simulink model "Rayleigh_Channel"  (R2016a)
settings: Solver=ode3  StartTime=0.0  StopTime=6  FixedStep=1/5000000  RelTol=1e-3
libraries: commchan3 x1

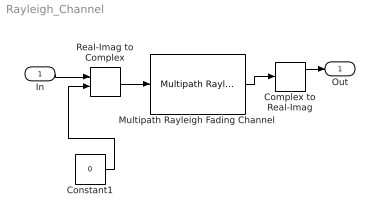
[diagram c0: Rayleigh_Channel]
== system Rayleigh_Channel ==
  In : Inport
  Complex to Real-Imag : ComplexToRealImag
  Constant1 : Constant  Value=0  SampleTime=1/5000000
  Multipath Rayleigh Fading Channel : commchan3/Multipath Rayleigh Fading Channel  maxDopplerShift=1  spectrumType=Jakes  sigmaGaussian=1/sqrt(2)  coeffRounded=[1 -1.72 0.785]  freqMinMaxRJakes=[0 1]  freqMinMaxAJakes=[0 1]  sigmaGaussian1=1/sqrt(2)  sigmaGaussian2=1/sqrt(2)  centerFreqGaussian1=0.0  centerFreqGaussian2=0.0  gainGaussian1=0.5  gainGaussian2=0.5  coeffBell=9  dopplerSpectrum=doppler.jakes  pathDelays=0  avgPathGaindB=-3  normalizePathGains=on  seed=73  enableProbe=0  openVisAtStart=off  outPathGains=off  outDelay=off
  Real-Imag to Complex : RealImagToComplex
  Out : Outport
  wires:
  In/1 -> Real-Imag to Complex/1
  Complex to Real-Imag/2 -> ?
  Complex to Real-Imag/1 -> Out/1
  Constant1/1 -> Real-Imag to Complex/2
  Multipath Rayleigh Fading Channel/1 -> Complex to Real-Imag/1
  Real-Imag to Complex/1 -> Multipath Rayleigh Fading Channel/1
